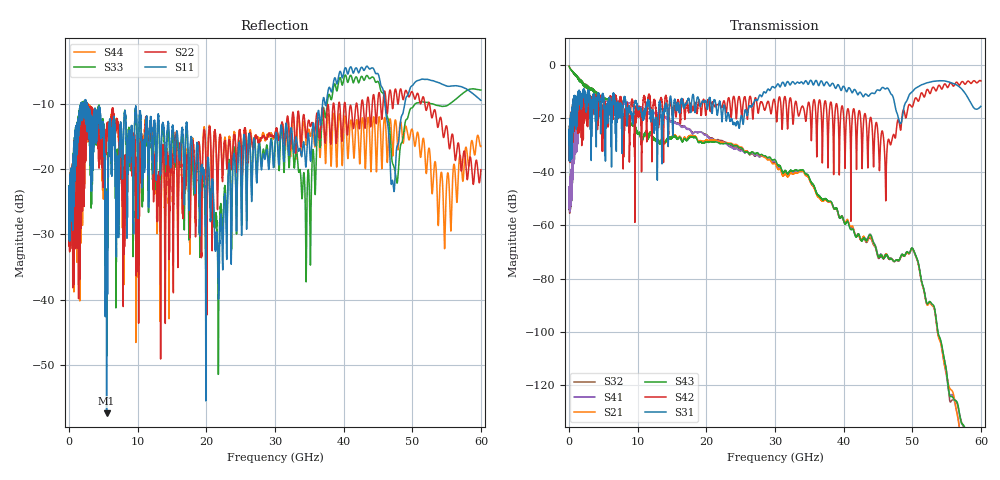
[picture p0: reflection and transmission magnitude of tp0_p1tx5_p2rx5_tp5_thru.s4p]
! 100G CR Analysis
! File: tp0_p1tx5_p2rx5_tp5_thru
! Description: 2m Cu Cable, OSFP, TP0-TP5
! Port Mapping
! Port1 -- P1TX5N
! Port2 -- P2RX5N
! Port3 -- P1TX5P
! Port4 -- P2RX5P
# GHz S MA R 50.00
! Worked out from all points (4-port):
!   6000 points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, 10 MHz to 60 GHz, reference 50 ohm
!   strongest paths, dB at 10 MHz, 15.01 GHz, 30.01 GHz, 45.01 GHz, 60 GHz:
!     S31: -28.0, -18.7, -8.6, -9.4, -15.5
!     S42: -27.9, -17.3, -14.1, -26.1, -6.0
!     S43: -0.5, -27.1, -35.5, -71.7, -156.7
!     S21: -0.5, -26.9, -37.0, -71.8, -155.9
!     S41: -46.1, -21.1, -36.1, -71.3, -158.4
!     S32: -46.3, -20.9, -36.4, -72.1, -162.9
!   lowest |S11| = -57.4 dB at 5.47 GHz (marker M1), VSWR 1.00, Z = 50 - j0.127 ohm
!   |S11| at or under -10 dB: start of sweep to 1.699 GHz; 2.565 GHz to 36.93 GHz (34.36 GHz wide, 174 % of centre); 46.04 GHz to 48.9 GHz (2.861 GHz wide, 6.03 % of centre)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
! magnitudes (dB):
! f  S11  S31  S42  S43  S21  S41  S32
! 10 MHz  -23.8  -28.0  -27.9  -0.5  -0.5  -46.1  -46.3
! 1.65 GHz  -10.4  -10.7  -11.5  -6.4  -6.4  -18.2  -18.0
! 5.47 GHz  -57.4  -18.8  -17.7  -12.7  -12.8  -13.3  -13.2
! 21.62 GHz  -31.7  -18.7  -14.8  -29.0  -28.4  -28.4  -28.0
! 36.5 GHz  -12.3  -7.1  -13.1  -49.3  -50.0  -49.7  -49.6
! 46.16 GHz  -11.4  -8.9  -47.8  -71.1  -70.9  -70.8  -71.2
! 60 GHz  -9.5  -15.5  -6.0  -156.7  -155.9  -158.4  -162.9
